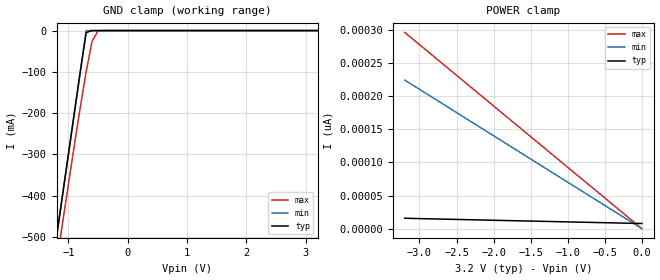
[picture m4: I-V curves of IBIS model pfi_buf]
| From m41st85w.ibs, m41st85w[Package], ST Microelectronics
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|   Model pfi_buf
[Model]   pfi_buf
Model_type   Input
Vinl =   0.3000V
Vinh =   0.7000V
C_comp   3.5600pF   3.4900pF   3.6100pF
[Temperature Range]   27.0000   85.0000   -40.0000
[Voltage Range]   3.2000V   2.7000V   3.6000V
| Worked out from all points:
|   GND clamp passes 1 mA (typ) near -0.62 V on its own axis
[GND_clamp]
| voltage   I(typ)   I(min)   I(max)
-3.2V     -2.5A      -2.5A      -2.534A
-1.2V     -500mA     -500mA     -563.9mA
-1.1V     -400mA     -400mA     -467.7mA
-900mV    -200mA     -200mA     -278.2mA
-800mV    -100mA     -100mA     -186.3mA
-700mV    -4.751mA   -78.61uA   -98.9mA
-600mV    -123.9uA   -4.74uA    -25.84mA
-500mV    -3.322uA   -522.7nA   -628.6uA
3.2V      7.737pA    8.397nA    7.561nA
[POWER_clamp]
| voltage   I(typ)   I(min)   I(max)
-3.2V     15.71pA    224.4pA    296.3pA
-2.9V     14.94pA    203.4pA    268.6pA
-1.9V     12.43pA    133.3pA    175.9pA
0V        7.769pA    0A         0A
